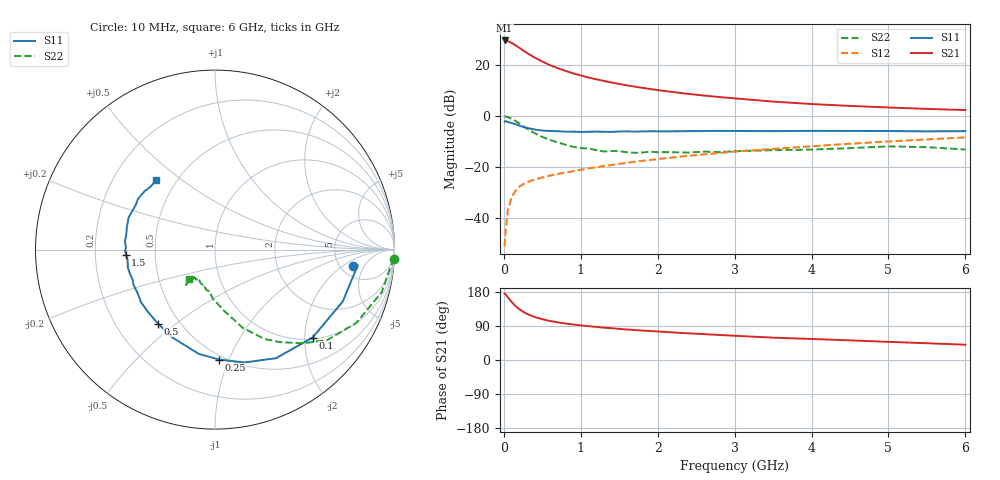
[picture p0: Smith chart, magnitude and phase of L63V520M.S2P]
!  INFINEON TECHNOLOGIES Small Signal Semiconductors
! BFR380L3 , Si-NPN RF-Transistor in TSLP-3-1
!  Vce=3.5 V,  Ic=20 mA
! Common Emitter S-Parameters:  07. March 2005
#  GHz  S  MA  R  50
! f  S11  S21  S12  S22
! GHz  Mag  Ang  Mag  Ang  Mag  Ang  Mag  Ang
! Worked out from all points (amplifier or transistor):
!   36 points, 10 MHz to 6 GHz, reference 50 ohm
!   highest |S21| = 29.7 dB at 10 MHz (marker M1)
!   |S21| within 3 dB of that: start of sweep to 206.6 MHz
!   unconditionally stable (mu >= 1): 1.98 GHz to 4.771 GHz
!   at 250 MHz: K = 0.34, MSG = 26.3 dB, |S12| = -26.7 dB
!   at 1.4 GHz: K = 0.93, MSG = 16.2 dB, |S12| = -19.2 dB
!   at 6 GHz: K = 0.97, MSG = 5.4 dB, |S12| = -8.4 dB
!   S11 on the Smith chart (normalised r, x): 10 MHz: 6.43, -2.91; 100 MHz: 1.04, -2.19; 250 MHz: 0.47, -0.92; 500 MHz: 0.38, -0.43; 1.5 GHz: 0.34, -0.03; 6 GHz: 0.39, +0.40
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0.01  0.7721 -6.8  30.51 175.2  0.0028 86.8  0.9991 -2.9
0.02  0.7997 -6.3  30.34 174.4  0.0049 81.6  0.9813 -5.9
0.05  0.7683 -22.1  29.56 165.9  0.0137 80.6  0.9588 -14.3
0.1  0.732 -42.0  27.33 153.5  0.0251 71.7  0.8871 -27.4
0.15  0.6942 -60.6  24.69 142.7  0.0341 64.3  0.8028 -38.9
0.2  0.6499 -75.4  21.93 134.2  0.0409 59.6  0.7154 -46.9
0.25  0.6132 -87.8  19.5 127.5  0.046 55.6  0.6308 -54.8
0.3  0.5878 -98.9  17.33 121.8  0.0502 53.7  0.5706 -60.9
0.4  0.5445 -115.8  14.09 113.4  0.057 51.9  0.4618 -70.6
0.5  0.5207 -127.7  11.77 107.6  0.0623 51.2  0.3905 -76.2
0.6  0.5097 -137.5  9.991 102.9  0.0679 51.2  0.3423 -81.9
0.7  0.5057 -144.4  8.725 99.4  0.0732 52.8  0.3035 -87.0
0.9  0.4946 -156.9  6.895 93.7  0.0825 54.7  0.2498 -95.6
1.1  0.4927 -164.3  5.731 89.2  0.0939 56.6  0.2308 -101.5
1.5  0.4983 -176.7  4.27 82.1  0.1157 59.5  0.2058 -111.6
1.8  0.5001 176.6  3.586 77.7  0.1323 60.9  0.1929 -117.1
2.2  0.5022 169.2  2.963 72.7  0.1548 61.7  0.1955 -121.1
2.8  0.5134 159.5  2.369 66.1  0.1888 62.7  0.1965 -128.5
3.5  0.5068 150.6  1.925 59.0  0.2273 61.6  0.2144 -128.8
4.5  0.5114 143.9  1.585 51.8  0.2864 61.0  0.2353 -129.3
5.5  0.5016 135.7  1.385 44.2  0.3485 58.0  0.2454 -129.6
6  0.5068 130.4  1.313 40.4  0.3813 56.1  0.2209 -131.1
